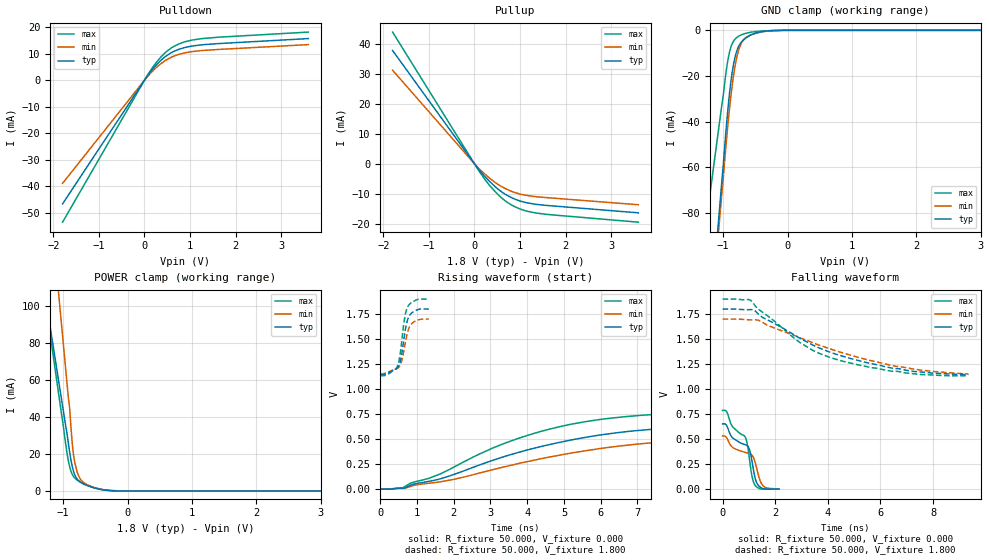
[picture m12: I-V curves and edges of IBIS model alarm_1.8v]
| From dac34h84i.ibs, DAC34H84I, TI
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[Model]   alarm_1.8v
Model_type 3-state
Vref=0.000E+00
Rref=1.000E+06
Cref=0.000E+00
Vmeas=9.000E-01
C_comp   6.290E-13   5.890E-13   6.690E-13
[Voltage Range]   1.800E+00   1.700E+00   1.900E+00
[POWER Clamp Reference]   1.800E+00   1.700E+00   1.900E+00
[GND Clamp Reference]   0.000E+00   0.000E+00   0.000E+00
[Pullup Reference]   1.800E+00   1.700E+00   1.900E+00
[Pulldown Reference]   0.000E+00   0.000E+00   0.000E+00
[Temperature Range] 25   125   -40
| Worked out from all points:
|   slope of the pulldown table from 0 to 0.27 V, typ, clamps not added: 45.6 ohm
|   slope of the pullup table from 0 to 0.27 V, typ, clamps not added: 54.8 ohm
|   GND clamp passes 1 mA (typ) near -0.47 V on its own axis
|   POWER clamp passes 1 mA (typ) near -0.45 V on its own axis
|   rising waveform, R_fixture 50.000, V_fixture 0.000: 20-80 % time 3.77ns typ, 4.29ns min, 3.27ns max; typ from 0 V to 0.652 V
|   falling waveform, R_fixture 50.000, V_fixture 0.000: 20-80 % time 870ps typ, 1.05ns min, 732ps max; typ from 0.652 V to 0 V
|   rising waveform, R_fixture 50.000, V_fixture 1.800: 20-80 % time 181ps typ, 197ps min, 170ps max; typ from 1.15 V to 1.8 V
|   falling waveform, R_fixture 50.000, V_fixture 1.800: 20-80 % time 3.42ns typ, 3.84ns min, 2.82ns max; typ from 1.8 V to 1.15 V
[GND Clamp]
-1.8V     -328.7mA   -322.1mA   -197.3mA
-1.02V    -65.95mA   -71.35mA   -32.57mA
-940mV    -38.74mA   -45.46mA   -15.36mA
-920mV    -32.7mA    -39.5mA    -12.02mA
-880mV    -22.5mA    -28.84mA   -7.352mA
-820mV    -12.26mA   -16.44mA   -3.98mA
-760mV    -7.071mA   -8.724mA   -2.578mA
-700mV    -4.644mA   -4.77mA    -1.784mA
-620mV    -2.857mA   -2.709mA   -1.148mA
-480mV    -1.075mA   -1.159mA   -490.5uA
-260mV    -173.3uA   -200.5uA   -106.3uA
3.6V      0A         0A         0A
[Power Clamp]
-1.8V     222mA      379.6mA    231.2mA
-1.02V    48.49mA    88.18mA    40.38mA
-920mV    26.11mA    50.82mA    16.48mA
-900mV    21.28mA    45.26mA    13.24mA
-860mV    13.47mA    26.21mA    9.068mA
-840mV    10.76mA    19.8mA     7.859mA
-820mV    8.766mA    15.59mA    6.999mA
-780mV    6.293mA    10.03mA    5.834mA
-700mV    4.052mA    5.069mA    4.276mA
-440mV    932.9uA    1.089mA    1.116mA
-120mV    0A         0A         0A
3.6V      0A         0A         0A
[Pullup]
-1.8V     37.98mA    31.37mA    44.14mA
120mV     -2.343mA   -1.92mA    -2.846mA
320mV     -5.701mA   -4.66mA    -7.03mA
540mV     -8.745mA   -7.128mA   -10.64mA
680mV     -10.23mA   -8.304mA   -12.46mA
820mV     -11.37mA   -9.256mA   -13.84mA
1V        -12.45mA   -10.12mA   -15.12mA
1.34V     -13.53mA   -10.99mA   -16.43mA
3.6V      -16.42mA   -13.71mA   -19.56mA
[Pulldown]
-1.8V     -46.56mA   -38.86mA   -53.48mA
80mV      1.966mA    1.636mA    2.274mA
280mV     6.106mA    5.077mA    7.112mA
480mV     9.176mA    7.651mA    10.74mA
600mV     10.48mA    8.749mA    12.28mA
760mV     11.66mA    9.756mA    13.69mA
1.04V     12.85mA    10.77mA    15.1mA
1.24V     13.29mA    11.15mA    15.62mA
3.6V      15.68mA    13.41mA    18.13mA
[Rising Waveform]
R_fixture = 50.000
V_fixture = 0.000
V_fixture_min = 0.000
V_fixture_max = 0.000
|  time   V(typ)   V(min)   V(max)
0s        0V         0V         0V
610ps     8.331mV    8.242mV    13.94mV
820ps     39.74mV    26.5mV     59.5mV
1.63ns    103mV      73.29mV    151.7mV
3.42ns    330.8mV    226.5mV    463.1mV
4.31ns    420.2mV    299mV      570.9mV
5.19ns    490.8mV    360.1mV    648.6mV
6.09ns    546.9mV    411.2mV    701.7mV
7.39ns    598.3mV    463.2mV    745mV
11.14ns   651.7mV    531.6mV    784.9mV
[Falling Waveform]
R_fixture = 50.000
V_fixture = 0.000
V_fixture_min = 0.000
V_fixture_max = 0.000
|  time   V(typ)   V(min)   V(max)
0s        651.7mV    531.6mV    784.9mV
160ps     632.7mV    511.2mV    772mV
380ps     512.3mV    416.6mV    622.8mV
870ps     442.6mV    365.2mV    515.3mV
950ps     429.4mV    359.7mV    434mV
1.04ns    378.2mV    353.5mV    262.1mV
1.12ns    275.6mV    338.7mV    124.6mV
1.24ns    106.8mV    264.7mV    35.92mV
1.52ns    5.227mV    37.76mV    -1.752mV
2.14ns    0V         0V         0V
[Rising Waveform]
R_fixture = 50.000
V_fixture = 1.800
V_fixture_min = 1.700
V_fixture_max = 1.900
|  time   V(typ)   V(min)   V(max)
0s        1.146V     1.152V     1.133V
200ps     1.158V     1.169V     1.146V
470ps     1.214V     1.208V     1.231V
510ps     1.237V     1.222V     1.282V
560ps     1.301V     1.257V     1.403V
670ps     1.567V     1.439V     1.725V
760ps     1.709V     1.589V     1.831V
840ps     1.756V     1.647V     1.863V
940ps     1.781V     1.677V     1.884V
1.32ns    1.8V       1.7V       1.9V
[Falling Waveform]
R_fixture = 50.000
V_fixture = 1.800
V_fixture_min = 1.700
V_fixture_max = 1.900
|  time   V(typ)   V(min)   V(max)
0s        1.8V       1.7V       1.9V
1.05ns    1.795V     1.692V     1.89V
1.21ns    1.786V     1.693V     1.842V
1.37ns    1.747V     1.688V     1.797V
2.95ns    1.507V     1.512V     1.464V
3.5ns     1.431V     1.456V     1.378V
4.27ns    1.352V     1.386V     1.301V
6.48ns    1.207V     1.233V     1.177V
7.98ns    1.159V     1.177V     1.141V
9.34ns    1.146V     1.152V     1.133V
[Ramp]
dV/dt_r   3.9031E-01/3.7675E-09   3.1871E-01/4.2841E-09   4.6746E-01/3.2656E-09
dV/dt_f   3.9249E-01/3.4144E-09   3.2885E-01/3.8422E-09   4.5993E-01/2.8128E-09
R_load = 50
